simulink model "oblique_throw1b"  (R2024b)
settings: Solver=VariableStepAuto  StartTime=0.0  StopTime=3  RelTol=1e-3

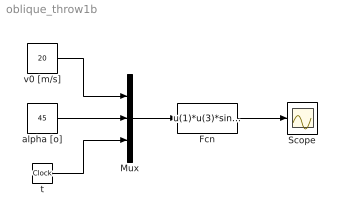
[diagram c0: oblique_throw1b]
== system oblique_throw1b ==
  Fcn : Fcn  Expr=u(1)*u(3)*sin(pi/180*u(2))-9.81*u(3)^2/2
  Mux : Mux  Inputs=3
  Scope : Scope
  alpha [o] : Constant  Value=45
  t : Clock
  v0 [m/s] : Constant  Value=20
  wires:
  v0 [m/s]/1 -> Mux/1
  alpha [o]/1 -> Mux/2
  t/1 -> Mux/3
  Mux/1 -> Fcn/1
  Fcn/1 -> Scope/1
